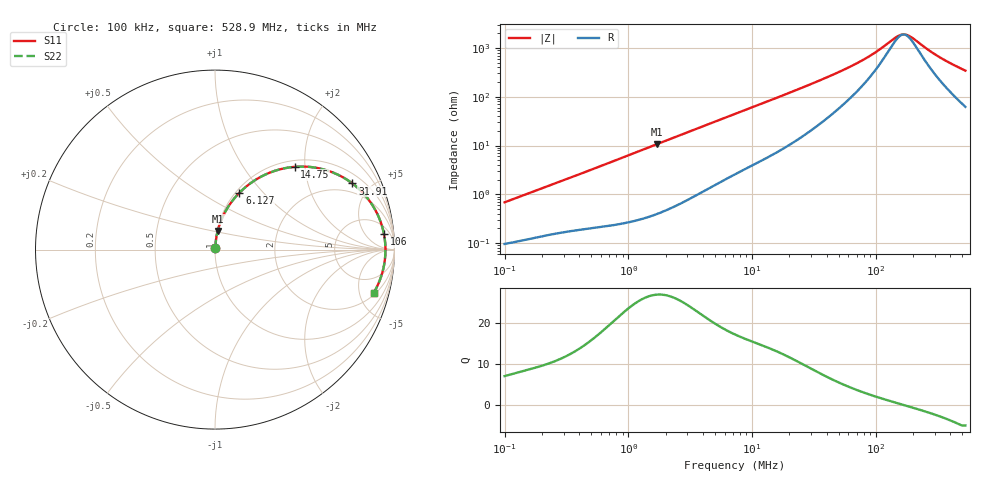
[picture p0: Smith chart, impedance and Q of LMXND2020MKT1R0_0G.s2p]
! LMXND2020MKT1R0_0G  S-PARAMETER MODEL  ( General Type )
! Model Generated by TAIYO YUDEN Corporation (https://www.yuden.co.jp/en/)
! Version 1.0
! TAIYO YUDEN Control No. 191023NI43SB-FBB
! Copyright(c) 2019 TAIYO YUDEN CO.,LTD. All Rights Reserved.
! Product Description (link to TY-COMPAS)
! https://ds.yuden.co.jp/TYCOMPAS/or/detail?pn=LMXND2020MKT1R0N0G&u=M
! Products Name : Inductors
! Characteristics :
!  Inductance : 1.0 uH , SRF(min) : -Hz , DC Resistance(max) : 0.084 Ohm
!  Rated Current : Saturation :1900 mA , Temp Rise : 1700 mA (40 degC)
!  Case Size : 2.0 x 2.0 / 0.079 x 0.079 [mm/inch] , Thickness : 1.2 / 0.047 [mm/inch]
!  (Conditions: Temperature = 25 degC , DC Bias Current/Voltage = 0A / 0V)
! External Node Assignments :
!  1  o---GGG---o  2
! GND o---------o GND
! Frequency Range : 0.1MHz  -  528.887669MHz  [ 402 STEP ]
# MHz S RI R 50
! Freq[MHz].  S11 Real  S11 Imag  S21 Real  S21 Imag  S12 Real  S12 Imag  S22 Real  S22 Imag
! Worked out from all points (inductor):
!   401 points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, 100 kHz to 528.9 MHz, reference 50 ohm
!   read as one part in series: L = 1.07 uH near 104.4 kHz
!   highest Q = 27 at 1.693 MHz (marker M1), where L = 995 nH
!   self-resonance near 167.6 MHz
!   S11 on the Smith chart (normalised r, x): 100 kHz: 1.00, +0.01; 6.127 MHz: 1.04, +0.75; 14.75 MHz: 1.13, +1.77; 31.91 MHz: 1.46, +3.87; 106 MHz: 10, +16; 528.9 MHz: 2.24, -6.74
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0.1  0.00101 0.00677  0.999 -0.00677  0.999 -0.00677  0.00101 0.00677
0.420401  0.00261 0.0267  0.9974 -0.0267  0.9974 -0.0267  0.00261 0.0267
1.693207  0.0149 0.1039  0.9851 -0.1039  0.9851 -0.1039  0.0149 0.1039
1.767367  0.016 0.1083  0.984 -0.1083  0.984 -0.1083  0.016 0.1083
3.585124  0.0554 0.2078  0.9446 -0.2078  0.9446 -0.2078  0.0554 0.2078
6.126528  0.1365 0.3172  0.8635 -0.3172  0.8635 -0.3172  0.1365 0.3172
7.430023  0.184 0.3593  0.816 -0.3593  0.816 -0.3593  0.184 0.3593
10.24746  0.2895 0.4222  0.7105 -0.4222  0.7105 -0.4222  0.2895 0.4222
14.75228  0.4442 0.4612  0.5558 -0.4612  0.5558 -0.4612  0.4442 0.4612
20.78709  0.6012 0.4477  0.3988 -0.4477  0.3988 -0.4477  0.6012 0.4477
30.5735  0.752 0.3784  0.248 -0.3784  0.248 -0.3784  0.752 0.3784
31.91258  0.7658 0.3683  0.2342 -0.3683  0.2342 -0.3683  0.7658 0.3683
44.01372  0.8489 0.2874  0.1511 -0.2874  0.1511 -0.2874  0.8489 0.2874
63.36231  0.9054 0.1967  0.0946 -0.1967  0.0946 -0.1967  0.9054 0.1967
83.72214  0.9296 0.134  0.0704 -0.134  0.0704 -0.134  0.9296 0.134
105.9822  0.9415 0.0858  0.0585 -0.0858  0.0585 -0.0858  0.9415 0.0858
128.5312  0.947 0.0489  0.053 -0.0489  0.053 -0.0489  0.947 0.0489
155.8778  0.9495 0.0133  0.0505 -0.0133  0.0505 -0.0133  0.9495 0.0133
166.23  0.9497 0.00154  0.0503 -0.00154  0.0503 -0.00154  0.9497 0.00154
181.1102  0.9496 -0.0141  0.0504 0.0141  0.0504 0.0141  0.9496 -0.0141
323.0502  0.9329 -0.1262  0.0671 0.1262  0.0671 0.1262  0.9329 -0.1262
528.8877  0.8842 -0.241  0.1158 0.241  0.1158 0.241  0.8842 -0.241
